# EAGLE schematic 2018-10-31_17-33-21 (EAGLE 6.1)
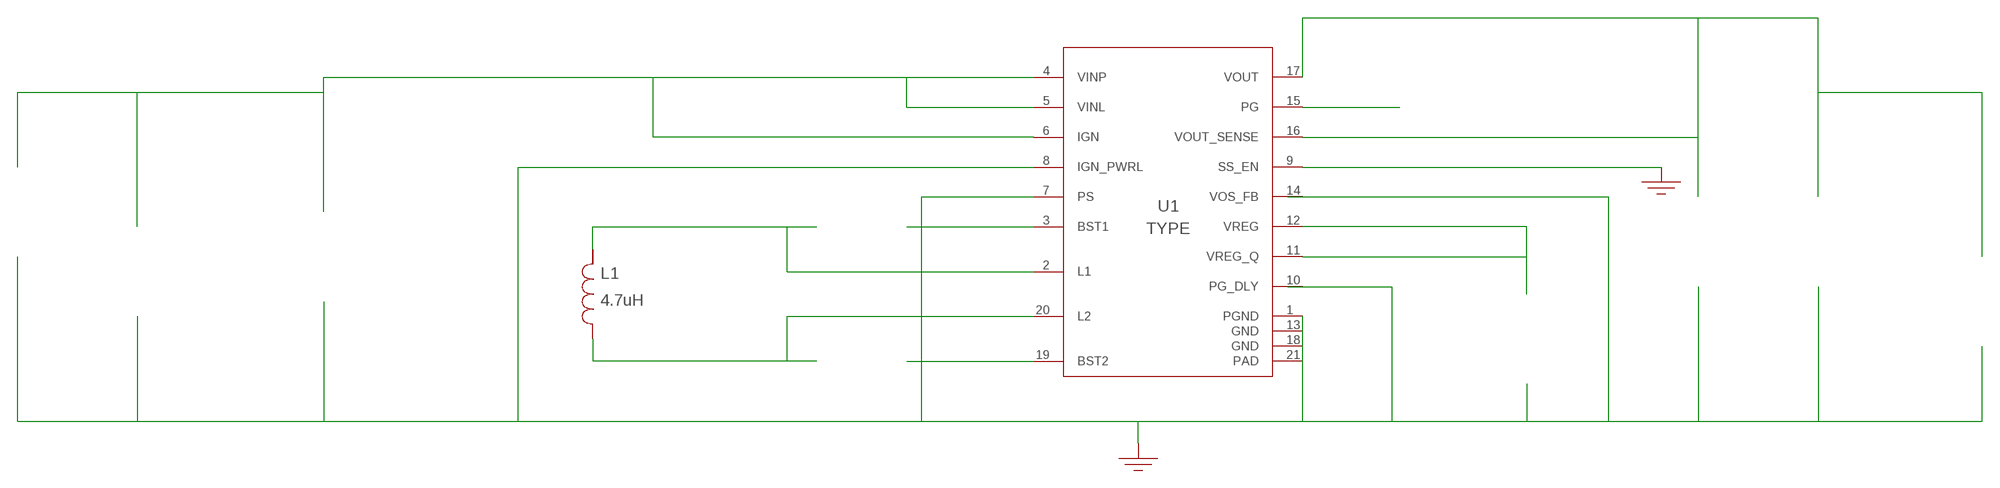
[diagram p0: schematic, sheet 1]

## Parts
CBST1  100nF  C0603C104Z3VACTUC0603C104Z3VACTU  [0603]  (not placed on a sheet)
CBST2  100nF  GRM155R71A104KA01DGRM155R71A104KA01D  [0402]  (not placed on a sheet)
CIN  22uF  C2012X5R1V226M125ACC2012X5R1V226M125AC  [0805]  (not placed on a sheet)
CINX  470nF  GMK212BJ474KG-TGMK212BJ474KG-T  [0805]  (not placed on a sheet)
CO_SENSE  100nF  C2012X7R1H104K085AAC2012X7R1H104K085AA  [0805]  (not placed on a sheet)
COUT  22uF  C2012X5R1V226M125ACC2012X5R1V226M125AC  [0805]  (not placed on a sheet)
CVREG  4.7uF  GRM155R61A475MEAADGRM155R61A475MEAAD  [0402]  (not placed on a sheet)
GND9  WB_GND  WB_GNDWB_GND  [WB_GND]
GND10  WB_GND  WB_GNDWB_GND  [WB_GND]
IOUT  WB_CURRENT_LOAD  WB_CURRENT_LOADWB_CURRENT_LOAD  [WB_CURRENT_LOAD]  (not placed on a sheet)
L1  4.7uH  XAL5030-472MEBXAL5030-472MEB  [XAL5030]
RPG  100k  ERJ-6ENF1003VERJ-6ENF1003V  [0805]  (not placed on a sheet)
U1  TPS55165QPWPRQ1  TPS55165QPWPRQ1TPS55165QPWPRQ1  [PWP0020P_N]
VIN  WB_BATTERY  WB_BATTERYWB_BATTERY  [WB_BATTERY]  (not placed on a sheet)

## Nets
0: Cin.2@2 Cinx.2@2 Co_sense.2@2 Cout.2@2 Cvreg.2@2 GND9.1 GND10.1 Iout.-@2 U1.1(PGND) U1.7(PS) U1.8(IGN_PWRL) U1.9(SS_EN) U1.10(PG_DLY) U1.13(GND) U1.14(VOS_FB) U1.18(GND) U1.21(PAD) Vin.-@2
1: Cbst2.2@2 U1.19(BST2)
2: Cbst1.2@2 U1.3(BST1)
3: Rpg.2@2 U1.15(PG)
5: Cin.1@1 Cinx.1@1 U1.4(VINP) U1.5(VINL) U1.6(IGN) Vin.+@1
6: Cbst2.1@1 L1.1 U1.20(L2)
7: Cbst1.1@1 L1.2 U1.2(L1)
8: Co_sense.1@1 Cout.1@1 Iout.+@1 Rpg.1@1 U1.16(VOUT_SENSE) U1.17(VOUT)
10: Cvreg.1@1 U1.11(VREG_Q) U1.12(VREG)
Unconnected: CBST1.1 CBST1.2 CBST2.1 CBST2.2 CIN.1 CIN.2 CINX.1 CINX.2 CO_SENSE.1 CO_SENSE.2 COUT.1 COUT.2 CVREG.1 CVREG.2 IOUT.1(+) IOUT.2(-) RPG.1 RPG.2 VIN.1(+) VIN.2(-)

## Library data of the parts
CBST1 = AcceleratedDesigns_Lib:C0603C104Z3VACTU; Cap: 1.0E-7; ESR: 0.0; IRMS: 0.0; Manufacturer_Name: Kemet; Manufacturer_Part_Number: C0603C104Z3VACTU; VDC: 25.0; Vendor: Kemet
CBST2 = AcceleratedDesigns_Lib:GRM155R71A104KA01D; Cap: 1.0E-7; ESR: 0.0; IRMS: 0.0; Manufacturer_Name: MuRata; Manufacturer_Part_Number: GRM155R71A104KA01D; VDC: 10.0; Vendor: MuRata
CIN COUT = AcceleratedDesigns_Lib:C2012X5R1V226M125AC; Cap: 2.2E-5; Datasheet_URL: https://product.tdk.com/en/search/capacitor/ceramic/mlcc/info?part%5Fno%3DC2012X5R1V226M125AC; ESR: 0.00205; IRMS: 4.55587; Manufacturer_Name: TDK; Manufacturer_Part_Number: C2012X5R1V226M125AC; VDC: 35.0; Vendor: TDK
CINX = AcceleratedDesigns_Lib:GMK212BJ474KG-T; Cap: 4.7E-7; ESR: 0.0; IRMS: 0.0; Manufacturer_Name: Taiyo Yuden; Manufacturer_Part_Number: GMK212BJ474KG-T; VDC: 35.0; Vendor: Taiyo Yuden
CO_SENSE = AcceleratedDesigns_Lib:C2012X7R1H104K085AA; Cap: 1.0E-7; Datasheet_URL: https://product.tdk.com/en/search/capacitor/ceramic/mlcc/info?part%5Fno%3DC2012X7R1H104K085AA; ESR: 0.02619; IRMS: 1.29514; Manufacturer_Name: TDK; Manufacturer_Part_Number: C2012X7R1H104K085AA; VDC: 50.0; Vendor: TDK
CVREG = AcceleratedDesigns_Lib:GRM155R61A475MEAAD; Cap: 4.7E-6; Datasheet_URL: http://search.murata.co.jp/Ceramy/image/img/A01X/G101/ENG/GRM155R61A475MEAA%2D01.pdf; ESR: 0.0; IRMS: 0.0; Manufacturer_Name: MuRata; Manufacturer_Part_Number: GRM155R61A475MEAAD; VDC: 10.0; Vendor: MuRata
GND9 GND10 = AcceleratedDesigns_Lib:WB_GND; Manufacturer_Name: WB_GND; Manufacturer_Part_Number: WB_GND; PowerPortType: POWER_GROUND; Value: Value
IOUT = AcceleratedDesigns_Lib:WB_CURRENT_LOAD; Manufacturer_Name: WB_CURRENT_LOAD; Manufacturer_Part_Number: WB_CURRENT_LOAD; PowerPortType: POWER_GROUND; Value: Value
L1 = AcceleratedDesigns_Lib:XAL5030-472MEB; DCR: 0.04; IDC: 5.9; L: 4.7E-6; Manufacturer_Name: Coilcraft; Manufacturer_Part_Number: XAL5030-472MEB; Vendor: Coilcraft
RPG = AcceleratedDesigns_Lib:ERJ-6ENF1003V; Manufacturer_Name: Panasonic; Manufacturer_Part_Number: ERJ-6ENF1003V; Power: 0.125; Resistance: 100000.0; Tolerance: 1.0; Vendor: Panasonic
U1 = AcceleratedDesigns_Lib:TPS55165QPWPRQ1; Manufacturer: Texas Instruments; Manufacturer_Name: Texas Instruments; Manufacturer_Part_Number: TPS55165QPWPRQ1; PartNumber: TPS55165PWPQ1; RefDes: RefDes; TYPE: TYPE; Value: Value
VIN = AcceleratedDesigns_Lib:WB_BATTERY; Manufacturer_Name: WB_BATTERY; Manufacturer_Part_Number: WB_BATTERY; PowerPortType: POWER_GROUND; Value: Value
